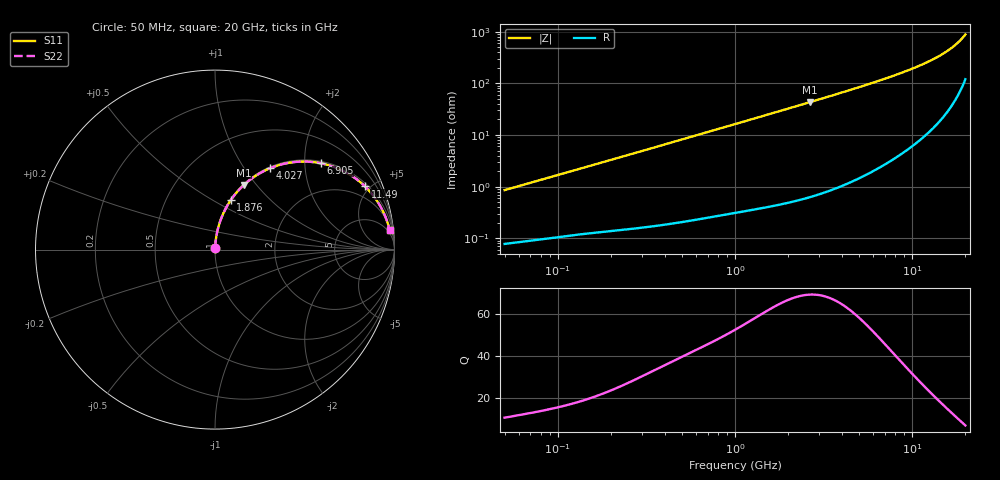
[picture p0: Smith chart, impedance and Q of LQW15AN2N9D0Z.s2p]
!Murata Part Number: LQW15AN2N9D0Z
!These Parameters are Measured in Series Mode Connection
!  o--[Z]--o
!Port1  Port2
!  o-------o
!Freq. Start=50[MHz] Stop=20[GHz], 401[Steps]
# Hz S RI R 50
!Freq.(Hz) S11(Real) S11(Imag) S21(Real) S21(Imag) S12(Real) S12(Imag) S22(Real) S22(Imag)
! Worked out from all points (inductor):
!   401 points, 50 MHz to 20 GHz, reference 50 ohm
!   read as one part in series: L = 2.7 nH near 51.52 MHz
!   highest Q = 68.9 at 2.647 GHz (marker M1), where L = 2.59 nH
!   S11 on the Smith chart (normalised r, x): 50 MHz: 1.00, +0.02; 1.876 GHz: 1.01, +0.61; 4.027 GHz: 1.02, +1.33; 6.905 GHz: 1.05, +2.40; 11.49 GHz: 1.18, +4.67; 20 GHz: 3, +17
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5e7  0.000851 0.00851  0.9991 -0.00851  0.9991 -0.00851  0.000851 0.00851
1.364002e8  0.00171 0.0226  0.9983 -0.0226  0.9983 -0.0226  0.00171 0.0226
3.721004e8  0.00543 0.0604  0.9946 -0.0604  0.9946 -0.0604  0.00543 0.0604
6.285508e8  0.0126 0.1007  0.9874 -0.1007  0.9874 -0.1007  0.0126 0.1007
1e9  0.0285 0.157  0.9715 -0.157  0.9715 -0.157  0.0285 0.157
1.411297e9  0.0529 0.2156  0.9471 -0.2156  0.9471 -0.2156  0.0529 0.2156
1.875929e9  0.0881 0.2759  0.9119 -0.2759  0.9119 -0.2759  0.0881 0.2759
2.647493e9  0.1602 0.3596  0.8398 -0.3596  0.8398 -0.3596  0.1602 0.3596
2.728004e9  0.1684 0.3671  0.8316 -0.3671  0.8316 -0.3671  0.1684 0.3671
3.314454e9  0.2308 0.414  0.7692 -0.414  0.7692 -0.414  0.2308 0.414
4.026975e9  0.3092 0.4545  0.6908 -0.4545  0.6908 -0.4545  0.3092 0.4545
5.352748e9  0.4493 0.4886  0.5507 -0.4886  0.5507 -0.4886  0.4493 0.4886
6.125241e9  0.5226 0.4898  0.4774 -0.4898  0.4774 -0.4898  0.5226 0.4898
6.905011e9  0.5887 0.4814  0.4113 -0.4814  0.4113 -0.4814  0.5887 0.4814
7.442007e9  0.6296 0.4715  0.3704 -0.4715  0.3704 -0.4715  0.6296 0.4715
9.316812e9  0.745 0.4216  0.255 -0.4216  0.255 -0.4216  0.745 0.4216
1.149051e10  0.8362 0.3517  0.1638 -0.3517  0.1638 -0.3517  0.8362 0.3517
1.354865e10  0.8931 0.2855  0.1069 -0.2855  0.1069 -0.2855  0.8931 0.2855
1.573793e10  0.9329 0.2196  0.0671 -0.2196  0.0671 -0.2196  0.9329 0.2196
1.774144e10  0.9564 0.1644  0.0436 -0.1644  0.0436 -0.1644  0.9564 0.1644
1.940974e10  0.9694 0.1221  0.0306 -0.1221  0.0306 -0.1221  0.9694 0.1221
2e10  0.9728 0.1078  0.0272 -0.1078  0.0272 -0.1078  0.9728 0.1078
